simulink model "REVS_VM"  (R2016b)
settings: Solver=ode3  StartTime=REVS.sim_start_time_secs  StopTime=Inf  FixedStep=REVS.sim_step_time_secs  MaxStep=REVS.sim_step_time_secs  EnableMultiTasking=on
StopFcn:
  | postproc_datalog;
  | postproc_audit;
  | postproc_result;
model workspace (MATLAB code in the model file):
  other statements: REVS_setup_variants
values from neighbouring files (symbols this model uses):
  accessory = class_accessory_data    [class_test_data.m]
  battery = class_battery_data    [class_accessory_data.m]    (also in class_REVS_electric.m = class_REVS_battery)
  brake = struct(	'max_torque_Nm',[], 						'proportion_norm',1.0, 						'inertia_kgm2',0.0)    [class_REVS_drive_axle.m]
  engine = class_engine_data    [class_test_data.m]
  final_drive = struct(	'gear_ratio',[], 								'efficiency_norm',[], 								'inertia_kgm2',[] )    [class_REVS_drive_axle.m]
  gear = class_REVS_gearbox    [class_REVS_AT_transmission.m]
  tire = struct(	'radius_m',[], 						'rolling_resistance_coefficient',0, 						'vehicle_weight_norm',1.0,  						'wheel_slip_torque_Nm',[],  						'inertia_kgm2',0.0)    [class_REVS_drive_axle.m]
  torque_converter = class_REVS_torque_converter    [class_REVS_AT_transmission.m]
  transmission = class_transmission_data    [class_test_data.m]
  vehicle = class_vehicle_data    [class_test_data.m]
undefined symbols (not defined in the file or in its folder): alternator, ambient, controls, convert, DelayTimeSecs, drive_cycle, driver, electric, gear_strategy, InitialCondition, InitialValue, LoadSource, LookupStructure, MultiplyPosInputs, Normalize, NumPhases, REVS, SpeedSource, starter, tableshift, UpperSaturationLimit, Value, VerboseLevel, VerboseSignal
libraries: simulink x153
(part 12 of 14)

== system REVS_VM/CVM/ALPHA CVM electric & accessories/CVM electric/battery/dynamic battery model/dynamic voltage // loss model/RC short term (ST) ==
  bus_in : Inport
  Add2 : Sum  Inputs=+-
  Bus Selector : BusSelector  OutputSignals=pack_curr_A
  Cp short term : Subsystem
  Integrator : Integrator
  Product4 : Product  Inputs=*/
  Product5 : Product  Inputs=*/
  Rp short term : Subsystem
  to datalog with base name : Subsystem
  to datalog with base name1 : Subsystem
  to datalog with base name2 : Subsystem
  RC_ST_V : Outport
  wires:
  Rp short term/1(Rp_ST_Ohm) -> to datalog with base name1/1(Var), Product5/2
  Bus Selector/1 -> Add2/1  "<pack_curr_A>"
  Integrator/1 -> RC_ST_V/1, to datalog with base name/1(Var), Product5/1
  Product4/1 -> Integrator/1
  Product5/1 -> Add2/2  "I ST"
  Add2/1 -> Product4/1
  Cp short term/1(Cp_ST_Farad) -> to datalog with base name2/1(Var), Product4/2
  bus_in/1 -> Cp short term/1(bus_in), Bus Selector/1, Rp short term/1(bus_in)

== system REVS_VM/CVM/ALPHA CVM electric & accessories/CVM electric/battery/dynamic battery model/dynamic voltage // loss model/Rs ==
  bus_in : Inport
  Bus Selector1 : BusSelector  OutputSignals=pack_curr_A
  Product1 : Product
  Rs charge : Subsystem
  Rs discharge : Subsystem
  Switch : Switch  Criteria=u2 > Threshold
  to datalog with base name : Subsystem
  to datalog with base name1 : Subsystem
  Rs_V : Outport
  Rs_dis_Ohm : Outport  Port=2
  Rs_chg_Ohm : Outport  Port=3
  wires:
  Product1/1 -> Rs_V/1, to datalog with base name/1(Var)
  Switch/1 -> Product1/2, to datalog with base name1/1(Var)
  Rs discharge/1(out) -> Switch/1, Rs_dis_Ohm/1
  Rs charge/1(out) -> Rs_chg_Ohm/1, Switch/3
  Bus Selector1/1 -> Product1/1, Switch/2  "<pack_curr_A>"
  bus_in/1 -> Rs discharge/1(bus), Rs charge/1(bus), Bus Selector1/1

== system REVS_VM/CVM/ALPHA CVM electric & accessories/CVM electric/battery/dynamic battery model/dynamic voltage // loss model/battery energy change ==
  Var : Inport
  Compare To Constant : simulink/Logic and Bit Operations/Compare To Constant  relop=>=  const=1  OutDataTypeStr=boolean
  Constant : Constant  Value=VerboseSignal
  Subsystem : Subsystem
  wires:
  Constant/1 -> Compare To Constant/1
  Compare To Constant/1 -> Subsystem/Enable
  Var/1 -> Subsystem/1(In1)

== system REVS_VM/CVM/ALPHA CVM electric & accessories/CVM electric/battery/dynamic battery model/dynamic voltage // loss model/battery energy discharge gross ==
  Var : Inport
  Compare To Constant : simulink/Logic and Bit Operations/Compare To Constant  relop=>=  const=1  OutDataTypeStr=boolean
  Constant : Constant  Value=VerboseSignal
  Subsystem : Subsystem
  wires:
  Constant/1 -> Compare To Constant/1
  Compare To Constant/1 -> Subsystem/Enable
  Var/1 -> Subsystem/1(In1)

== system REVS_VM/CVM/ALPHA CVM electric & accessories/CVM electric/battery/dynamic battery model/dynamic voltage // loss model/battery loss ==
  Var : Inport
  Compare To Constant : simulink/Logic and Bit Operations/Compare To Constant  relop=>=  const=1  OutDataTypeStr=boolean
  Constant : Constant  Value=VerboseSignal
  Subsystem : Subsystem
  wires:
  Constant/1 -> Compare To Constant/1
  Compare To Constant/1 -> Subsystem/Enable
  Var/1 -> Subsystem/1(In1)

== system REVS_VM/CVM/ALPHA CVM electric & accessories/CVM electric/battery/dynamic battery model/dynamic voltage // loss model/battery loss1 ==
  Var : Inport
  Compare To Constant : simulink/Logic and Bit Operations/Compare To Constant  relop=>=  const=1  OutDataTypeStr=boolean
  Constant : Constant  Value=VerboseSignal
  Subsystem : Subsystem
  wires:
  Constant/1 -> Compare To Constant/1
  Compare To Constant/1 -> Subsystem/Enable
  Var/1 -> Subsystem/1(In1)

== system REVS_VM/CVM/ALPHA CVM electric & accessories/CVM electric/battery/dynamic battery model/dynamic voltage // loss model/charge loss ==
  charge_eff_norm : Inport
  pack_curr_A : Inport  Port=2
  OCV_V : Inport  Port=3
  Compare To Zero : simulink/Logic and Bit Operations/Compare To Zero  relop=<=  OutDataTypeStr=uint8
  Constant2 : Constant
  Data Type Conversion : DataTypeConversion  OutDataTypeStr=double
  Gain1 : Gain  Gain=-1
  Product7 : Product  Inputs=4  OutDataTypeStr=double
  Sum : Sum  Inputs=|+-
  chg_loss_pwr_W : Outport
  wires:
  Gain1/1 -> Product7/3
  pack_curr_A/1 -> Gain1/1, Compare To Zero/1
  OCV_V/1 -> Product7/4
  charge_eff_norm/1 -> Sum/2
  Data Type Conversion/1 -> Product7/2
  Constant2/1 -> Sum/1
  Compare To Zero/1 -> Data Type Conversion/1
  Sum/1 -> Product7/1
  Product7/1 -> chg_loss_pwr_W/1

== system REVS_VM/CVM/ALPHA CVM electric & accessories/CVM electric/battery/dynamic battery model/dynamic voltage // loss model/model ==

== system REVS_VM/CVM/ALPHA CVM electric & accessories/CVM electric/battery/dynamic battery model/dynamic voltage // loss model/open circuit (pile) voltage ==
  bus_in : Inport
  Add : Sum
  Bus Selector : BusSelector  OutputSignals=pack_curr_A
  Gain : Gain  Gain=0.5
  OCV charge dynamic : Subsystem
  OCV discharge dynamic : Subsystem
  Switch : Switch  Criteria=u2 ~= 0
  Switch1 : Switch
  to datalog with base name : Subsystem
  use average : Constant  Value=battery.use_average_open_circuit_Volts
  OCV_V : Outport
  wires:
  Switch/1 -> OCV_V/1, to datalog with base name/1(Var)
  OCV discharge dynamic/1(out) -> Add/1, Switch1/1
  OCV charge dynamic/1(out) -> Add/2, Switch1/3
  Switch1/1 -> Switch/3
  use average/1 -> Switch/2
  bus_in/1 -> OCV discharge dynamic/1(bus), OCV charge dynamic/1(bus), Bus Selector/1
  Add/1 -> Gain/1
  Gain/1 -> Switch/1
  Bus Selector/1 -> Switch1/2  "<pack_curr_A>"

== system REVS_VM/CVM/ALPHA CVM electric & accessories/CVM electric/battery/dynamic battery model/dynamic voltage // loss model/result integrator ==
  in : Inport
  Data Type Conversion : DataTypeConversion  OutDataTypeStr=double
  Integrator1 : Integrator  UpperSaturationLimit=Inf  LowerSaturationLimit=0  ZeroCross=off
  Integrator2 : Integrator  UpperSaturationLimit=Inf  LowerSaturationLimit=0  ZeroCross=off
  Phase To Workspace : ToWorkspace  VariableName=result__phase_battery_delta_kJ  SampleTime=-1
  Product1 : Product  Multiplication=Matrix(*)
  Reshape : Reshape
  Total To Workspace : ToWorkspace  VariableName=result__total_battery_delta_kJ  SampleTime=-1
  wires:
  Reshape/1 -> Integrator1/1, Product1/1
  Data Type Conversion/1 -> Reshape/1
  Integrator2/1 -> Phase To Workspace/1
  [REVS_phase_flag] -> Product1/2
  Product1/1 -> Integrator2/1
  Integrator1/1 -> Total To Workspace/1
  in/1 -> Data Type Conversion/1

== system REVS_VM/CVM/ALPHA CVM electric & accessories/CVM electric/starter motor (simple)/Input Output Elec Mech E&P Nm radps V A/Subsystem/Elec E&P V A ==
  volts_V : Inport
  curr_A : Inport  Port=2
  Compare To Constant : simulink/Logic and Bit Operations/Compare To Constant  relop=>=  const=1  OutDataTypeStr=boolean
  Constant : Constant  Value=VerboseSignal
  Subsystem : Subsystem
  pos_kJ : Outport
  neg_kJ : Outport  Port=2
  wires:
  volts_V/1 -> Subsystem/1(volts_V)
  curr_A/1 -> Subsystem/2(curr_A)
  Subsystem/1(pos_kJ) -> pos_kJ/1
  Subsystem/2(neg_kJ) -> neg_kJ/1
  Compare To Constant/1 -> Subsystem/Enable
  Constant/1 -> Compare To Constant/1

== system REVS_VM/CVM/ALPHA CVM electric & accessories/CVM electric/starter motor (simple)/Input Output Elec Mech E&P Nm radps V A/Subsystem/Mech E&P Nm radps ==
  " trq_Nm" : Inport
  spd_radps : Inport  Port=2
  iner_kgm2 : Inport  Port=3
  Compare To Constant : simulink/Logic and Bit Operations/Compare To Constant  relop=>=  const=1  OutDataTypeStr=boolean
  Constant : Constant  Value=VerboseSignal
  Subsystem : Subsystem
  pos_kJ : Outport
  neg_kJ : Outport  Port=2
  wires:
  " trq_Nm"/1 -> Subsystem/1(" trq_Nm")
  spd_radps/1 -> Subsystem/2(spd_radps)
  iner_kgm2/1 -> Subsystem/3(iner_kgm2)
  Compare To Constant/1 -> Subsystem/Enable
  Subsystem/1(pos_kJ) -> pos_kJ/1
  Subsystem/2(neg_kJ) -> neg_kJ/1
  Constant/1 -> Compare To Constant/1

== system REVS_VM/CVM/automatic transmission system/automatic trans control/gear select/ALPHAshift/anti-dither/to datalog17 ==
  Var : Inport
  Constant : Constant  Value=VerboseSignal
  Constant1 : Constant  Value=VerboseLevel
  Relational Operator : RelationalOperator  OutDataTypeStr=boolean  ZeroCross=off
  Subsystem : Subsystem
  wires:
  Constant1/1 -> Relational Operator/2
  Constant/1 -> Relational Operator/1
  Relational Operator/1 -> Subsystem/Enable
  Var/1 -> Subsystem/1(In1)

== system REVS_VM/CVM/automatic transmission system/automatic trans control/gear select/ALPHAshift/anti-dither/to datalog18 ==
  Var : Inport
  Constant : Constant  Value=VerboseSignal
  Constant1 : Constant  Value=VerboseLevel
  Relational Operator : RelationalOperator  OutDataTypeStr=boolean  ZeroCross=off
  Subsystem : Subsystem
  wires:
  Constant1/1 -> Relational Operator/2
  Constant/1 -> Relational Operator/1
  Relational Operator/1 -> Subsystem/Enable
  Var/1 -> Subsystem/1(In1)

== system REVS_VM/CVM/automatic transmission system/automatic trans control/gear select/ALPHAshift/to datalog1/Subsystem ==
  In1 : Inport
  Enable : EnablePort
  To Workspace : ToWorkspace  VariableName=datalog__ALPHAshift__desired_gear_num  SampleTime=-1
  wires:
  In1/1 -> To Workspace/1

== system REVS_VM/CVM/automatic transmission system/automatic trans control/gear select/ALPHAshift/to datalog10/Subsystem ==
  In1 : Inport
  Enable : EnablePort
  To Workspace : ToWorkspace  VariableName=datalog__ALPHAshift__kickdown_timer  SampleTime=-1
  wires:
  In1/1 -> To Workspace/1

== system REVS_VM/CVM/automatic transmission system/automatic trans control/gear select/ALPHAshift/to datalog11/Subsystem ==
  In1 : Inport
  Enable : EnablePort
  To Workspace : ToWorkspace  VariableName=datalog__ALPHAshift__kickdown_ratio  SampleTime=-1
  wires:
  In1/1 -> To Workspace/1

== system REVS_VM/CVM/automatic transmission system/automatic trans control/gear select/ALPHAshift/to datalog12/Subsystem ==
  In1 : Inport
  Enable : EnablePort
  To Workspace : ToWorkspace  VariableName=datalog__ALPHAshift__shift_delay_timer  SampleTime=-1
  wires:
  In1/1 -> To Workspace/1

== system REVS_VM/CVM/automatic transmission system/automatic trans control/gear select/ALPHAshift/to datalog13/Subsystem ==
  In1 : Inport
  Enable : EnablePort
  To Workspace : ToWorkspace  VariableName=datalog__ALPHAshift__in_gear_timer  SampleTime=-1
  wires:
  In1/1 -> To Workspace/1

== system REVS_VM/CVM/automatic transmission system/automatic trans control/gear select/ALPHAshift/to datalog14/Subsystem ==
  In1 : Inport
  Enable : EnablePort
  To Workspace : ToWorkspace  VariableName=datalog__ALPHAshift__gear_avail_torque_Nm  SampleTime=-1
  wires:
  In1/1 -> To Workspace/1

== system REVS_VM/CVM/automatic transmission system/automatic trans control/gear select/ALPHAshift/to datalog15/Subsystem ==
  In1 : Inport
  Enable : EnablePort
  To Workspace : ToWorkspace  VariableName=datalog__ALPHAshift__gear_speed_radps  SampleTime=-1
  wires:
  In1/1 -> To Workspace/1

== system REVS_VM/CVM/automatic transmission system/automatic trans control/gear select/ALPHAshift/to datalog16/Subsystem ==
  In1 : Inport
  Enable : EnablePort
  To Workspace : ToWorkspace  VariableName=datalog__ALPHAshift__gear_torque_Nm  SampleTime=-1
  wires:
  In1/1 -> To Workspace/1

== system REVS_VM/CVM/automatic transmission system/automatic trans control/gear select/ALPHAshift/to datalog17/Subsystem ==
  In1 : Inport
  Enable : EnablePort
  To Workspace : ToWorkspace  VariableName=datalog__ALPHAshift__gear_cost  SampleTime=-1
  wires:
  In1/1 -> To Workspace/1

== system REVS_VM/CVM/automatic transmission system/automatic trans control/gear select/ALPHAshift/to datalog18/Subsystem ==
  In1 : Inport
  Enable : EnablePort
  To Workspace : ToWorkspace  VariableName=datalog__ALPHAshift__kickdown_disability_code  SampleTime=-1
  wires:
  In1/1 -> To Workspace/1

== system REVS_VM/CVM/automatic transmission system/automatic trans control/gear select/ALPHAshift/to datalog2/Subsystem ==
  In1 : Inport
  Enable : EnablePort
  To Workspace : ToWorkspace  VariableName=datalog__ALPHAshift__shift_reason  SampleTime=-1
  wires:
  In1/1 -> To Workspace/1

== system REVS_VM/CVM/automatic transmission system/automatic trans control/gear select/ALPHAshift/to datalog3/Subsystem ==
  In1 : Inport
  Enable : EnablePort
  To Workspace : ToWorkspace  VariableName=datalog__ALPHAshift__disability_code  SampleTime=-1
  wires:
  In1/1 -> To Workspace/1

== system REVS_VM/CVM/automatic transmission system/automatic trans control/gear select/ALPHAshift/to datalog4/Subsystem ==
  In1 : Inport
  Enable : EnablePort
  To Workspace : ToWorkspace  VariableName=datalog__ALPHAshift__current_gear_num  SampleTime=-1
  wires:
  In1/1 -> To Workspace/1

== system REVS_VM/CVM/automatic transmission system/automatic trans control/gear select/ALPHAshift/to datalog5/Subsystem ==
  In1 : Inport
  Enable : EnablePort
  To Workspace : ToWorkspace  VariableName=datalog__ALPHAshift__gear_available  SampleTime=-1
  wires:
  In1/1 -> To Workspace/1

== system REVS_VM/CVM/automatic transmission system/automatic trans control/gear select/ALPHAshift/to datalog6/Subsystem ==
  In1 : Inport
  Enable : EnablePort
  To Workspace : ToWorkspace  VariableName=datalog__ALPHAshift__shift_type  SampleTime=-1
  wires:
  In1/1 -> To Workspace/1

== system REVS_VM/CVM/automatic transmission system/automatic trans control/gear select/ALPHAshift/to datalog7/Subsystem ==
  In1 : Inport
  Enable : EnablePort
  To Workspace : ToWorkspace  VariableName=datalog__ALPHAshift__better_fuel_gear  SampleTime=-1
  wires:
  In1/1 -> To Workspace/1

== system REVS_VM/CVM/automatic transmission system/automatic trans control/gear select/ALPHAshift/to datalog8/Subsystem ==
  In1 : Inport
  Enable : EnablePort
  To Workspace : ToWorkspace  VariableName=datalog__ALPHAshift__min_fuel_gear  SampleTime=-1
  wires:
  In1/1 -> To Workspace/1

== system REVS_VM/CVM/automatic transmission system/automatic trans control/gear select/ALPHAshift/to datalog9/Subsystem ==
  In1 : Inport
  Enable : EnablePort
  To Workspace : ToWorkspace  VariableName=datalog__ALPHAshift__desired_shift_reason  SampleTime=-1
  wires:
  In1/1 -> To Workspace/1

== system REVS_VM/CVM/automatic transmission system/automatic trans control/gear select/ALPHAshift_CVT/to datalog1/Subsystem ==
  In1 : Inport
  Enable : EnablePort
  To Workspace : ToWorkspace  VariableName=datalog__cvtshift__target_ratio  SampleTime=-1
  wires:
  In1/1 -> To Workspace/1

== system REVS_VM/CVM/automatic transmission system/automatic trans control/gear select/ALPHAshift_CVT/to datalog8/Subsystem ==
  In1 : Inport
  Enable : EnablePort
  To Workspace : ToWorkspace  VariableName=datalog__cvtshift__target_speed_radps  SampleTime=-1
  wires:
  In1/1 -> To Workspace/1

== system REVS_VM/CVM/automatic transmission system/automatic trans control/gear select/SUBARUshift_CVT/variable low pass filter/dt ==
  Clock : Clock
  Memory1 : Memory
  Sum : Sum  Inputs=|-+
  dt : Outport
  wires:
  Clock/1 -> Sum/2, Memory1/1
  Memory1/1 -> Sum/1
  Sum/1 -> dt/1

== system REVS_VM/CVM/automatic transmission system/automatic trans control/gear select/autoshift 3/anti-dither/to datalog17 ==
  Var : Inport
  Constant : Constant  Value=VerboseSignal
  Constant1 : Constant  Value=VerboseLevel
  Relational Operator : RelationalOperator  OutDataTypeStr=boolean  ZeroCross=off
  Subsystem : Subsystem
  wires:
  Constant1/1 -> Relational Operator/2
  Constant/1 -> Relational Operator/1
  Relational Operator/1 -> Subsystem/Enable
  Var/1 -> Subsystem/1(In1)

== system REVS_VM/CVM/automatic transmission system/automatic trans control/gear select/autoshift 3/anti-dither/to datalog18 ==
  Var : Inport
  Constant : Constant  Value=VerboseSignal
  Constant1 : Constant  Value=VerboseLevel
  Relational Operator : RelationalOperator  OutDataTypeStr=boolean  ZeroCross=off
  Subsystem : Subsystem
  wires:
  Constant1/1 -> Relational Operator/2
  Constant/1 -> Relational Operator/1
  Relational Operator/1 -> Subsystem/Enable
  Var/1 -> Subsystem/1(In1)

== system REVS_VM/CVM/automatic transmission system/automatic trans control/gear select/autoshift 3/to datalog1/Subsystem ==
  In1 : Inport
  Enable : EnablePort
  To Workspace : ToWorkspace  VariableName=datalog__autoshift3__desired_gear_num  SampleTime=-1
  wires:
  In1/1 -> To Workspace/1

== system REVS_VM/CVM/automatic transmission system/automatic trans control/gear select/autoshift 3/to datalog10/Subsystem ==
  In1 : Inport
  Enable : EnablePort
  To Workspace : ToWorkspace  VariableName=datalog__autoshift3__kickdown_timer  SampleTime=-1
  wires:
  In1/1 -> To Workspace/1

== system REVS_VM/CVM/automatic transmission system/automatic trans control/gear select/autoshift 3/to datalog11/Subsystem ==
  In1 : Inport
  Enable : EnablePort
  To Workspace : ToWorkspace  VariableName=datalog__autoshift3__kickdown_ratio  SampleTime=-1
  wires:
  In1/1 -> To Workspace/1

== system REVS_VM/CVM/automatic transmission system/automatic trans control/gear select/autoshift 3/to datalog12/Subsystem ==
  In1 : Inport
  Enable : EnablePort
  To Workspace : ToWorkspace  VariableName=datalog__autoshift3__shift_delay_timer  SampleTime=-1
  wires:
  In1/1 -> To Workspace/1

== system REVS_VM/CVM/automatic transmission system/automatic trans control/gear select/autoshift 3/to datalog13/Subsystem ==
  In1 : Inport
  Enable : EnablePort
  To Workspace : ToWorkspace  VariableName=datalog__autoshift3__in_gear_timer  SampleTime=-1
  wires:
  In1/1 -> To Workspace/1

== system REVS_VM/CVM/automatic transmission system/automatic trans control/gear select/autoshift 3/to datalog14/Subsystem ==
  In1 : Inport
  Enable : EnablePort
  To Workspace : ToWorkspace  VariableName=datalog__autoshift3__gear_avail_torque_Nm  SampleTime=-1
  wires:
  In1/1 -> To Workspace/1

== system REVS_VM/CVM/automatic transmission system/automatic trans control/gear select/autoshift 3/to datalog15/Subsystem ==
  In1 : Inport
  Enable : EnablePort
  To Workspace : ToWorkspace  VariableName=datalog__autoshift3__gear_speed_radps  SampleTime=-1
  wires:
  In1/1 -> To Workspace/1

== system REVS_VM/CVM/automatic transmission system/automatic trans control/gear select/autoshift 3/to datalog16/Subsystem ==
  In1 : Inport
  Enable : EnablePort
  To Workspace : ToWorkspace  VariableName=datalog__autoshift3__gear_torque_Nm  SampleTime=-1
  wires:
  In1/1 -> To Workspace/1

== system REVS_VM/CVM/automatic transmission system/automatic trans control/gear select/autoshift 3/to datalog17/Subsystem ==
  In1 : Inport
  Enable : EnablePort
  To Workspace : ToWorkspace  VariableName=datalog__autoshift3__gear_cost  SampleTime=-1
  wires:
  In1/1 -> To Workspace/1

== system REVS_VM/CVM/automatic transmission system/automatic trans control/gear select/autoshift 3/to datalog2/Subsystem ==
  In1 : Inport
  Enable : EnablePort
  To Workspace : ToWorkspace  VariableName=datalog__autoshift3__shift_reason  SampleTime=-1
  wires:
  In1/1 -> To Workspace/1

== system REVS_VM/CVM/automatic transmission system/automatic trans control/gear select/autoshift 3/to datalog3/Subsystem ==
  In1 : Inport
  Enable : EnablePort
  To Workspace : ToWorkspace  VariableName=datalog__autoshift3__disability_code  SampleTime=-1
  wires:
  In1/1 -> To Workspace/1

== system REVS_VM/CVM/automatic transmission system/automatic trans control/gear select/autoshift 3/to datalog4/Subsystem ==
  In1 : Inport
  Enable : EnablePort
  To Workspace : ToWorkspace  VariableName=datalog__autoshift3__current_gear_num  SampleTime=-1
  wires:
  In1/1 -> To Workspace/1

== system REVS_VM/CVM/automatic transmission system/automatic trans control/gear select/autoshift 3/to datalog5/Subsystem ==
  In1 : Inport
  Enable : EnablePort
  To Workspace : ToWorkspace  VariableName=datalog__autoshift3__gear_available  SampleTime=-1
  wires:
  In1/1 -> To Workspace/1

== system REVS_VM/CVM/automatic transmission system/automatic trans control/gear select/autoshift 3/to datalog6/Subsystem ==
  In1 : Inport
  Enable : EnablePort
  To Workspace : ToWorkspace  VariableName=datalog__autoshift3__shift_type  SampleTime=-1
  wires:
  In1/1 -> To Workspace/1

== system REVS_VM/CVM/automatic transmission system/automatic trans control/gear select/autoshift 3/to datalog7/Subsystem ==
  In1 : Inport
  Enable : EnablePort
  To Workspace : ToWorkspace  VariableName=datalog__autoshift3__better_fuel_gear  SampleTime=-1
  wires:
  In1/1 -> To Workspace/1

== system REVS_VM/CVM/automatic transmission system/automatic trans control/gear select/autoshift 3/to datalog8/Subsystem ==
  In1 : Inport
  Enable : EnablePort
  To Workspace : ToWorkspace  VariableName=datalog__autoshift3__min_fuel_gear  SampleTime=-1
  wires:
  In1/1 -> To Workspace/1

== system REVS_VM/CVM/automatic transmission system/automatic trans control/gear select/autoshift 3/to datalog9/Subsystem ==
  In1 : Inport
  Enable : EnablePort
  To Workspace : ToWorkspace  VariableName=datalog__autoshift3__desired_shift_reason  SampleTime=-1
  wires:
  In1/1 -> To Workspace/1

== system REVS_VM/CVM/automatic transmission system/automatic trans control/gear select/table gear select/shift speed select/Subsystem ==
  veh_spd_mps : Inport
  Axle Speed (rad/sec) : Product  Inputs=/*
  Non Zero : Saturate  UpperLimit=Inf  LowerLimit=eps  ZeroCross=off
  Tire Radius (m) : Constant  Value=vehicle.drive_axle1.tire.radius_m
  wheel_spd_radps : Outport
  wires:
  veh_spd_mps/1 -> Axle Speed (rad/sec)/2
  Non Zero/1 -> Axle Speed (rad/sec)/1
  Axle Speed (rad/sec)/1 -> wheel_spd_radps/1
  Tire Radius (m)/1 -> Non Zero/1

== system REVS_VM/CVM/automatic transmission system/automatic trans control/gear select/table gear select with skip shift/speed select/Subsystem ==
  veh_spd_mps : Inport
  Axle Speed (rad/sec) : Product  Inputs=/*
  Non Zero : Saturate  UpperLimit=Inf  LowerLimit=eps  ZeroCross=off
  Tire Radius (m) : Constant  Value=vehicle.drive_axle1.tire.radius_m
  wheel_spd_radps : Outport
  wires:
  veh_spd_mps/1 -> Axle Speed (rad/sec)/2
  Non Zero/1 -> Axle Speed (rad/sec)/1
  Axle Speed (rad/sec)/1 -> wheel_spd_radps/1
  Tire Radius (m)/1 -> Non Zero/1

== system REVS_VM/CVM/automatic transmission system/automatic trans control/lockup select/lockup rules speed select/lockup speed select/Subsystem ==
  veh_spd_mps : Inport
  Axle Speed (rad/sec) : Product  Inputs=/*
  Non Zero : Saturate  UpperLimit=Inf  LowerLimit=eps  ZeroCross=off
  Tire Radius (m) : Constant  Value=vehicle.drive_axle1.tire.radius_m
  wheel_spd_radps : Outport
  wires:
  veh_spd_mps/1 -> Axle Speed (rad/sec)/2
  Non Zero/1 -> Axle Speed (rad/sec)/1
  Axle Speed (rad/sec)/1 -> wheel_spd_radps/1
  Tire Radius (m)/1 -> Non Zero/1

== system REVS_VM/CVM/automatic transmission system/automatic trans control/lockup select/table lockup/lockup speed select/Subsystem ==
  veh_spd_mps : Inport
  Axle Speed (rad/sec) : Product  Inputs=/*
  Non Zero : Saturate  UpperLimit=Inf  LowerLimit=eps  ZeroCross=off
  Tire Radius (m) : Constant  Value=vehicle.drive_axle1.tire.radius_m
  wheel_spd_radps : Outport
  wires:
  veh_spd_mps/1 -> Axle Speed (rad/sec)/2
  Non Zero/1 -> Axle Speed (rad/sec)/1
  Axle Speed (rad/sec)/1 -> wheel_spd_radps/1
  Tire Radius (m)/1 -> Non Zero/1

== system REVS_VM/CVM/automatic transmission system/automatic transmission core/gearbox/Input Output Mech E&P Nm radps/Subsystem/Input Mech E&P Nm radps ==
  " trq_Nm" : Inport
  spd_radps : Inport  Port=2
  iner_kgm2 : Inport  Port=3
  Compare To Constant : simulink/Logic and Bit Operations/Compare To Constant  relop=>=  const=1  OutDataTypeStr=boolean
  Constant : Constant  Value=VerboseSignal
  Subsystem : Subsystem
  pos_kJ : Outport
  neg_kJ : Outport  Port=2
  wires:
  " trq_Nm"/1 -> Subsystem/1(" trq_Nm")
  spd_radps/1 -> Subsystem/2(spd_radps)
  iner_kgm2/1 -> Subsystem/3(iner_kgm2)
  Compare To Constant/1 -> Subsystem/Enable
  Subsystem/1(pos_kJ) -> pos_kJ/1
  Subsystem/2(neg_kJ) -> neg_kJ/1
  Constant/1 -> Compare To Constant/1

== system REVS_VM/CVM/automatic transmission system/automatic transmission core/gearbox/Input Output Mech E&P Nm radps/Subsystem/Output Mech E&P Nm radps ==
  " trq_Nm" : Inport
  spd_radps : Inport  Port=2
  iner_kgm2 : Inport  Port=3
  Compare To Constant : simulink/Logic and Bit Operations/Compare To Constant  relop=>=  const=1  OutDataTypeStr=boolean
  Constant : Constant  Value=VerboseSignal
  Subsystem : Subsystem
  pos_kJ : Outport
  neg_kJ : Outport  Port=2
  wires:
  " trq_Nm"/1 -> Subsystem/1(" trq_Nm")
  spd_radps/1 -> Subsystem/2(spd_radps)
  iner_kgm2/1 -> Subsystem/3(iner_kgm2)
  Compare To Constant/1 -> Subsystem/Enable
  Subsystem/1(pos_kJ) -> pos_kJ/1
  Subsystem/2(neg_kJ) -> neg_kJ/1
  Constant/1 -> Compare To Constant/1

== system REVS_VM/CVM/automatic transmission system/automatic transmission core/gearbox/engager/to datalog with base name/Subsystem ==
  Var : Inport
  Enable : EnablePort
  To Workspace : ToWorkspace  VariableName=datalog__gearbox__current_gear  SampleTime=-1
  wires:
  Var/1 -> To Workspace/1

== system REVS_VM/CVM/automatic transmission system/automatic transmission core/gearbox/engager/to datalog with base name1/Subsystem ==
  Var : Inport
  Enable : EnablePort
  To Workspace : ToWorkspace  VariableName=datalog__gearbox__gearbox__engage_norm  SampleTime=-1
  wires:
  Var/1 -> To Workspace/1

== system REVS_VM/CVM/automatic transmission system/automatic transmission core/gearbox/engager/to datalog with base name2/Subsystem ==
  Var : Inport
  Enable : EnablePort
  To Workspace : ToWorkspace  VariableName=datalog__gearbox__command_gear  SampleTime=-1
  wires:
  Var/1 -> To Workspace/1

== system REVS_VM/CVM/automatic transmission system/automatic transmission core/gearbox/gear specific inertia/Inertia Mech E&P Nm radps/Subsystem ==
  trq_Nm : Inport
  spd_radps : Inport  Port=2
  Enable : EnablePort  ZeroCross=off
  Mech Energy Nm radps : Subsystem  TreatAsAtomicUnit=on
  energy_to_workspace : ToWorkspace  VariableName=audit__mech__gearbox__inertia_spinup_loss_kJ  SampleTime=-1
  neg_energy_to_workspace : ToWorkspace  VariableName=audit__mech__gearbox__inertia_spinup_loss_neg_kJ  SampleTime=-1
  pos_energy_to_workspace : ToWorkspace  VariableName=audit__mech__gearbox__inertia_spinup_loss_pos_kJ  SampleTime=-1
  power_to_workspace : ToWorkspace  VariableName=audit__mech__gearbox__inertia_spinup_loss_kW  SampleTime=-1
  speed_to_workspace : ToWorkspace  VariableName=audit__mech__gearbox__inertia_spinup_loss_radps  SampleTime=-1
  torque_to_workspace : ToWorkspace  VariableName=audit__mech__gearbox__inertia_spinup_loss_Nm  SampleTime=-1
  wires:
  Mech Energy Nm radps/1("total_kJ ") -> energy_to_workspace/1
  Mech Energy Nm radps/4(pwr_kW) -> power_to_workspace/1
  Mech Energy Nm radps/2("pos_kJ ") -> pos_energy_to_workspace/1
  Mech Energy Nm radps/3(neg_kJ) -> neg_energy_to_workspace/1
  trq_Nm/1 -> torque_to_workspace/1, Mech Energy Nm radps/1(trq_Nm)
  spd_radps/1 -> speed_to_workspace/1, Mech Energy Nm radps/2(spd_radps)

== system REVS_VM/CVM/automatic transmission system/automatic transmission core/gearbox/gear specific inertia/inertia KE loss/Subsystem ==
  In1 : Inport
  Enable : EnablePort
  To Workspace : ToWorkspace  VariableName=audit__mech__gearbox__inertia_KE_loss_kJ  SampleTime=-1
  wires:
  In1/1 -> To Workspace/1

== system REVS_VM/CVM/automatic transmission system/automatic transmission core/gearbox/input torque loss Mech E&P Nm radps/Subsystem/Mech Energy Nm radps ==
  trq_Nm : Inport
  spd_radps : Inport  Port=2
  Gain : Gain  Gain=-1
  Integrator : Integrator  ZeroCross=off
  Integrator1 : Integrator  ZeroCross=off
  Integrator2 : Integrator  ZeroCross=off
  Mux : Mux  Inputs=2
  Neg : Fcn  Expr=u(1)*(u(1) <= 0)
  Pos : Fcn  Expr=u(1)*(u(1) >= 0)
  calc_Power_kW : Fcn  Expr=u(1)*u(2)/1000
  "total_kJ " : Outport
  "pos_kJ " : Outport  Port=2
  neg_kJ : Outport  Port=3
  pwr_kW : Outport  Port=4
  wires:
  calc_Power_kW/1 -> Pos/1, Neg/1, pwr_kW/1, Integrator/1
  Gain/1 -> neg_kJ/1
  Integrator1/1 -> "pos_kJ "/1
  Integrator2/1 -> Gain/1
  Neg/1 -> Integrator2/1
  Pos/1 -> Integrator1/1
  spd_radps/1 -> Mux/2
  trq_Nm/1 -> Mux/1
  Mux/1 -> calc_Power_kW/1
  Integrator/1 -> "total_kJ "/1

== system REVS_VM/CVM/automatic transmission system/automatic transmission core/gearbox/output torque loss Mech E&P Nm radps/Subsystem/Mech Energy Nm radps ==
  trq_Nm : Inport
  spd_radps : Inport  Port=2
  Gain : Gain  Gain=-1
  Integrator : Integrator  ZeroCross=off
  Integrator1 : Integrator  ZeroCross=off
  Integrator2 : Integrator  ZeroCross=off
  Mux : Mux  Inputs=2
  Neg : Fcn  Expr=u(1)*(u(1) <= 0)
  Pos : Fcn  Expr=u(1)*(u(1) >= 0)
  calc_Power_kW : Fcn  Expr=u(1)*u(2)/1000
  "total_kJ " : Outport
  "pos_kJ " : Outport  Port=2
  neg_kJ : Outport  Port=3
  pwr_kW : Outport  Port=4
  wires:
  calc_Power_kW/1 -> Pos/1, Neg/1, pwr_kW/1, Integrator/1
  Gain/1 -> neg_kJ/1
  Integrator1/1 -> "pos_kJ "/1
  Integrator2/1 -> Gain/1
  Neg/1 -> Integrator2/1
  Pos/1 -> Integrator1/1
  spd_radps/1 -> Mux/2
  trq_Nm/1 -> Mux/1
  Mux/1 -> calc_Power_kW/1
  Integrator/1 -> "total_kJ "/1

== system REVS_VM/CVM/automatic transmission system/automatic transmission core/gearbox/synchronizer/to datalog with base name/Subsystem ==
  Var : Inport
  Enable : EnablePort
  To Workspace : ToWorkspace  VariableName=datalog__gearbox__gear_synchronizer_lockup  SampleTime=-1
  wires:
  Var/1 -> To Workspace/1

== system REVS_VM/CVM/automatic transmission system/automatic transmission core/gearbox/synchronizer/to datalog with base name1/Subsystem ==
  Var : Inport
  Enable : EnablePort
  To Workspace : ToWorkspace  VariableName=datalog__gearbox__synchronizer_transmit_torque_Nm  SampleTime=-1
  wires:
  Var/1 -> To Workspace/1

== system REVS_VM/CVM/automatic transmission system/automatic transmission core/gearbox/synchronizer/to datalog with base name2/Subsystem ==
  Var : Inport
  Enable : EnablePort
  To Workspace : ToWorkspace  VariableName=datalog__gearbox__synchronizer_engage_torque_Nm  SampleTime=-1
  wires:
  Var/1 -> To Workspace/1

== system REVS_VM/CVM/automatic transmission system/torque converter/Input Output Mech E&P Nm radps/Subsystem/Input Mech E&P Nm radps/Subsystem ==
  " trq_Nm" : Inport
  spd_radps : Inport  Port=2
  iner_kgm2 : Inport  Port=3
  Enable : EnablePort  ZeroCross=off
  KE_to_workspace : ToWorkspace  VariableName=audit__mech__torque_converter__input_KE_kJ  SampleTime=-1
  Mech Energy Nm radps : Subsystem  TreatAsAtomicUnit=on
  Mult : Product  Inputs=**
  Square : Math  Operator=square
  energy_to_workspace : ToWorkspace  VariableName=audit__mech__torque_converter__input_kJ  SampleTime=-1
  inertia_to_workspace : ToWorkspace  VariableName=audit__mech__torque_converter__input_kgm2  SampleTime=-1
  neg_energy_to_workspace : ToWorkspace  VariableName=audit__mech__torque_converter__input_neg_kJ  SampleTime=-1
  one half : Gain  Gain=0.5/1000
  pos_energy_to_workspace : ToWorkspace  VariableName=audit__mech__torque_converter__input_pos_kJ  SampleTime=-1
  power_to_workspace : ToWorkspace  VariableName=audit__mech__torque_converter__input_kW  SampleTime=-1
  speed_to_workspace : ToWorkspace  VariableName=audit__mech__torque_converter__input_radps  SampleTime=-1
  torque_to_workspace : ToWorkspace  VariableName=audit__mech__torque_converter__input_Nm  SampleTime=-1
  pos_kJ : Outport  InitialOutput=0
  neg_kJ : Outport  Port=2  InitialOutput=0
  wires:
  Mult/1 -> one half/1
  Square/1 -> Mult/1
  one half/1 -> KE_to_workspace/1
  Mech Energy Nm radps/4(pwr_kW) -> power_to_workspace/1
  Mech Energy Nm radps/1("total_kJ ") -> energy_to_workspace/1
  iner_kgm2/1 -> inertia_to_workspace/1, Mult/2
  spd_radps/1 -> Mech Energy Nm radps/2(spd_radps), speed_to_workspace/1, Square/1
  " trq_Nm"/1 -> Mech Energy Nm radps/1(trq_Nm), torque_to_workspace/1
  Mech Energy Nm radps/2("pos_kJ ") -> pos_kJ/1, pos_energy_to_workspace/1
  Mech Energy Nm radps/3(neg_kJ) -> neg_energy_to_workspace/1, neg_kJ/1

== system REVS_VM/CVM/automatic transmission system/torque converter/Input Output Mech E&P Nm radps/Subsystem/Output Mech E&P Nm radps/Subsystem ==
  " trq_Nm" : Inport
  spd_radps : Inport  Port=2
  iner_kgm2 : Inport  Port=3
  Enable : EnablePort  ZeroCross=off
  KE_to_workspace : ToWorkspace  VariableName=audit__mech__torque_converter__output_KE_kJ  SampleTime=-1
  Mech Energy Nm radps : Subsystem  TreatAsAtomicUnit=on
  Mult : Product  Inputs=**
  Square : Math  Operator=square
  energy_to_workspace : ToWorkspace  VariableName=audit__mech__torque_converter__output_kJ  SampleTime=-1
  inertia_to_workspace : ToWorkspace  VariableName=audit__mech__torque_converter__output_kgm2  SampleTime=-1
  neg_energy_to_workspace : ToWorkspace  VariableName=audit__mech__torque_converter__output_neg_kJ  SampleTime=-1
  one half : Gain  Gain=0.5/1000
  pos_energy_to_workspace : ToWorkspace  VariableName=audit__mech__torque_converter__output_pos_kJ  SampleTime=-1
  power_to_workspace : ToWorkspace  VariableName=audit__mech__torque_converter__output_kW  SampleTime=-1
  speed_to_workspace : ToWorkspace  VariableName=audit__mech__torque_converter__output_radps  SampleTime=-1
  torque_to_workspace : ToWorkspace  VariableName=audit__mech__torque_converter__output_Nm  SampleTime=-1
  pos_kJ : Outport  InitialOutput=0
  neg_kJ : Outport  Port=2  InitialOutput=0
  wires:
  Mult/1 -> one half/1
  Square/1 -> Mult/1
  one half/1 -> KE_to_workspace/1
  Mech Energy Nm radps/4(pwr_kW) -> power_to_workspace/1
  Mech Energy Nm radps/1("total_kJ ") -> energy_to_workspace/1
  iner_kgm2/1 -> inertia_to_workspace/1, Mult/2
  spd_radps/1 -> Mech Energy Nm radps/2(spd_radps), speed_to_workspace/1, Square/1
  " trq_Nm"/1 -> Mech Energy Nm radps/1(trq_Nm), torque_to_workspace/1
  Mech Energy Nm radps/2("pos_kJ ") -> pos_kJ/1, pos_energy_to_workspace/1
  Mech Energy Nm radps/3(neg_kJ) -> neg_energy_to_workspace/1, neg_kJ/1

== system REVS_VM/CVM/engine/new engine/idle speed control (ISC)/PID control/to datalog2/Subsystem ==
  In1 : Inport
  Enable : EnablePort
  To Workspace : ToWorkspace  VariableName=datalog__engine__ISC_Ki_torque_Nm  SampleTime=-1
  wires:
  In1/1 -> To Workspace/1

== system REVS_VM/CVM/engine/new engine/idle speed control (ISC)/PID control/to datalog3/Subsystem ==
  In1 : Inport
  Enable : EnablePort
  To Workspace : ToWorkspace  VariableName=datalog__engine__ISC_Kp_torque_Nm  SampleTime=-1
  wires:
  In1/1 -> To Workspace/1

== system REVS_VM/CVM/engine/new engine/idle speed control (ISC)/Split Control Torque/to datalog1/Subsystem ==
  In1 : Inport
  Enable : EnablePort
  To Workspace : ToWorkspace  VariableName=datalog__engine__ISC_torque_Nm  SampleTime=-1
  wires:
  In1/1 -> To Workspace/1

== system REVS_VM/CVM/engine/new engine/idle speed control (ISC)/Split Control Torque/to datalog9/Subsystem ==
  In1 : Inport
  Enable : EnablePort
  To Workspace : ToWorkspace  VariableName=datalog__engine__ISC_est_slow_torque_Nm  SampleTime=-1
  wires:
  In1/1 -> To Workspace/1

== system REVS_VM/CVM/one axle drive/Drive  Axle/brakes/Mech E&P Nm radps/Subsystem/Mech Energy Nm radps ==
  trq_Nm : Inport
  spd_radps : Inport  Port=2
  Gain : Gain  Gain=-1
  Integrator : Integrator  ZeroCross=off
  Integrator1 : Integrator  ZeroCross=off
  Integrator2 : Integrator  ZeroCross=off
  Mux : Mux  Inputs=2
  Neg : Fcn  Expr=u(1)*(u(1) <= 0)
  Pos : Fcn  Expr=u(1)*(u(1) >= 0)
  calc_Power_kW : Fcn  Expr=u(1)*u(2)/1000
  "total_kJ " : Outport
  "pos_kJ " : Outport  Port=2
  neg_kJ : Outport  Port=3
  pwr_kW : Outport  Port=4
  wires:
  calc_Power_kW/1 -> Pos/1, Neg/1, pwr_kW/1, Integrator/1
  Gain/1 -> neg_kJ/1
  Integrator1/1 -> "pos_kJ "/1
  Integrator2/1 -> Gain/1
  Neg/1 -> Integrator2/1
  Pos/1 -> Integrator1/1
  spd_radps/1 -> Mux/2
  trq_Nm/1 -> Mux/1
  Mux/1 -> calc_Power_kW/1
  Integrator/1 -> "total_kJ "/1

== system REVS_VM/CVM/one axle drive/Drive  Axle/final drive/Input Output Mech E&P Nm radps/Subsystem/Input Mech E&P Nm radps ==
  " trq_Nm" : Inport
  spd_radps : Inport  Port=2
  iner_kgm2 : Inport  Port=3
  Compare To Constant : simulink/Logic and Bit Operations/Compare To Constant  relop=>=  const=1  OutDataTypeStr=boolean
  Constant : Constant  Value=VerboseSignal
  Subsystem : Subsystem
  pos_kJ : Outport
  neg_kJ : Outport  Port=2
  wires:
  " trq_Nm"/1 -> Subsystem/1(" trq_Nm")
  spd_radps/1 -> Subsystem/2(spd_radps)
  iner_kgm2/1 -> Subsystem/3(iner_kgm2)
  Compare To Constant/1 -> Subsystem/Enable
  Subsystem/1(pos_kJ) -> pos_kJ/1
  Subsystem/2(neg_kJ) -> neg_kJ/1
  Constant/1 -> Compare To Constant/1

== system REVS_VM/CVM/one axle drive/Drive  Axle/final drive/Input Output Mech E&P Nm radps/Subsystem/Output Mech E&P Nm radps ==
  " trq_Nm" : Inport
  spd_radps : Inport  Port=2
  iner_kgm2 : Inport  Port=3
  Compare To Constant : simulink/Logic and Bit Operations/Compare To Constant  relop=>=  const=1  OutDataTypeStr=boolean
  Constant : Constant  Value=VerboseSignal
  Subsystem : Subsystem
  pos_kJ : Outport
  neg_kJ : Outport  Port=2
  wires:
  " trq_Nm"/1 -> Subsystem/1(" trq_Nm")
  spd_radps/1 -> Subsystem/2(spd_radps)
  iner_kgm2/1 -> Subsystem/3(iner_kgm2)
  Compare To Constant/1 -> Subsystem/Enable
  Subsystem/1(pos_kJ) -> pos_kJ/1
  Subsystem/2(neg_kJ) -> neg_kJ/1
  Constant/1 -> Compare To Constant/1

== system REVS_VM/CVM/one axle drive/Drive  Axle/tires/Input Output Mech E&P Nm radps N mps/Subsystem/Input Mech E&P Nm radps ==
  " trq_Nm" : Inport
  spd_radps : Inport  Port=2
  iner_kgm2 : Inport  Port=3
  Compare To Constant : simulink/Logic and Bit Operations/Compare To Constant  relop=>=  const=1  OutDataTypeStr=boolean
  Constant : Constant  Value=VerboseSignal
  Subsystem : Subsystem
  pos_kJ : Outport
  neg_kJ : Outport  Port=2
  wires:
  Constant/1 -> Compare To Constant/1
  Subsystem/2(neg_kJ) -> neg_kJ/1
  Subsystem/1(pos_kJ) -> pos_kJ/1
  Compare To Constant/1 -> Subsystem/Enable
  iner_kgm2/1 -> Subsystem/3(iner_kgm2)
  spd_radps/1 -> Subsystem/2(spd_radps)
  " trq_Nm"/1 -> Subsystem/1(" trq_Nm")

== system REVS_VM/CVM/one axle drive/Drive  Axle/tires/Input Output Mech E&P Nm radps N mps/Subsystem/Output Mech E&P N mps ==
  force_N : Inport
  spd_mps : Inport  Port=2
  mass_kg : Inport  Port=3
  Compare To Constant : simulink/Logic and Bit Operations/Compare To Constant  relop=>=  const=1  OutDataTypeStr=boolean
  Constant : Constant  Value=VerboseSignal
  Subsystem : Subsystem
  pos_kJ : Outport
  neg_kJ : Outport  Port=2
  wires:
  Subsystem/2(neg_kJ) -> neg_kJ/1
  Subsystem/1(pos_kJ) -> pos_kJ/1
  force_N/1 -> Subsystem/1(force_N)
  spd_mps/1 -> Subsystem/2(spd_mps)
  mass_kg/1 -> Subsystem/3(mass_kg)
  Compare To Constant/1 -> Subsystem/Enable
  Constant/1 -> Compare To Constant/1

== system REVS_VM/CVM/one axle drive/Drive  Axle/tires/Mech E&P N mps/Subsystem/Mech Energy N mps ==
  force_N : Inport
  spd_mps : Inport  Port=2
  Gain : Gain  Gain=-1
  Integrator : Integrator  ZeroCross=off
  Integrator1 : Integrator  ZeroCross=off
  Integrator2 : Integrator  ZeroCross=off
  Mux : Mux  Inputs=2
  Neg : Fcn  Expr=u(1)*(u(1) <= 0)
  Pos : Fcn  Expr=u(1)*(u(1) >= 0)
  calc_Power_kW : Fcn  Expr=u(1)*u(2)/1000
  "total_kJ " : Outport
  "pos_kJ " : Outport  Port=2
  neg_kJ : Outport  Port=3
  pwr_kW : Outport  Port=4
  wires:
  calc_Power_kW/1 -> Pos/1, Neg/1, pwr_kW/1, Integrator/1
  Gain/1 -> neg_kJ/1
  Integrator1/1 -> "pos_kJ "/1
  Integrator2/1 -> Gain/1
  Neg/1 -> Integrator2/1
  Pos/1 -> Integrator1/1
  Integrator/1 -> "total_kJ "/1
  Mux/1 -> calc_Power_kW/1
  force_N/1 -> Mux/1
  spd_mps/1 -> Mux/2

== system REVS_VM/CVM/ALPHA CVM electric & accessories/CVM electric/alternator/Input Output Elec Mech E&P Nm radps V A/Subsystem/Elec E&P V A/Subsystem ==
  volts_V : Inport
  curr_A : Inport  Port=2
  Enable : EnablePort  ZeroCross=off
  Elec Energy V A : Subsystem  TreatAsAtomicUnit=on
  amps_to_workspace : ToWorkspace  VariableName=audit__elec__alternator__input_Amps  SampleTime=-1
  energy_to_workspace : ToWorkspace  VariableName=audit__elec__alternator__input_kJ  SampleTime=-1
  neg_energy_to_workspace : ToWorkspace  VariableName=audit__elec__alternator__input_neg_kJ  SampleTime=-1
  pos_energy_to_workspace : ToWorkspace  VariableName=audit__elec__alternator__input_pos_kJ  SampleTime=-1
  power_to_workspace : ToWorkspace  VariableName=audit__elec__alternator__input_kW  SampleTime=-1
  volts_to_workspace : ToWorkspace  VariableName=audit__elec__alternator__input_Volts  SampleTime=-1
  pos_kJ : Outport  InitialOutput=0
  neg_kJ : Outport  Port=2  InitialOutput=0
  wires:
  Elec Energy V A/3(neg_kJ) -> neg_kJ/1, neg_energy_to_workspace/1
  Elec Energy V A/4(pwr_kW) -> power_to_workspace/1
  Elec Energy V A/2("pos_kJ ") -> pos_kJ/1, pos_energy_to_workspace/1
  Elec Energy V A/1("total_kJ ") -> energy_to_workspace/1
  volts_V/1 -> volts_to_workspace/1, Elec Energy V A/1(volts_V)
  curr_A/1 -> amps_to_workspace/1, Elec Energy V A/2(curr_A)

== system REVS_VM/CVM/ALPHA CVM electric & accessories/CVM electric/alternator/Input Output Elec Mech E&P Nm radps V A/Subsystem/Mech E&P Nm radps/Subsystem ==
  " trq_Nm" : Inport
  spd_radps : Inport  Port=2
  iner_kgm2 : Inport  Port=3
  Enable : EnablePort  ZeroCross=off
  KE_to_workspace : ToWorkspace  VariableName=audit__mech__alternator__output_KE_kJ  SampleTime=-1
  Mech Energy Nm radps : Subsystem  TreatAsAtomicUnit=on
  Mult : Product  Inputs=**
  Square : Math  Operator=square
  energy_to_workspace : ToWorkspace  VariableName=audit__mech__alternator__output_kJ  SampleTime=-1
  inertia_to_workspace : ToWorkspace  VariableName=audit__mech__alternator__output_kgm2  SampleTime=-1
  neg_energy_to_workspace : ToWorkspace  VariableName=audit__mech__alternator__output_neg_kJ  SampleTime=-1
  one half : Gain  Gain=0.5/1000
  pos_energy_to_workspace : ToWorkspace  VariableName=audit__mech__alternator__output_pos_kJ  SampleTime=-1
  power_to_workspace : ToWorkspace  VariableName=audit__mech__alternator__output_kW  SampleTime=-1
  speed_to_workspace : ToWorkspace  VariableName=audit__mech__alternator__output_radps  SampleTime=-1
  torque_to_workspace : ToWorkspace  VariableName=audit__mech__alternator__output_Nm  SampleTime=-1
  pos_kJ : Outport  InitialOutput=0
  neg_kJ : Outport  Port=2  InitialOutput=0
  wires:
  Mult/1 -> one half/1
  Square/1 -> Mult/1
  one half/1 -> KE_to_workspace/1
  Mech Energy Nm radps/4(pwr_kW) -> power_to_workspace/1
  Mech Energy Nm radps/1("total_kJ ") -> energy_to_workspace/1
  iner_kgm2/1 -> inertia_to_workspace/1, Mult/2
  spd_radps/1 -> Mech Energy Nm radps/2(spd_radps), speed_to_workspace/1, Square/1
  " trq_Nm"/1 -> Mech Energy Nm radps/1(trq_Nm), torque_to_workspace/1
  Mech Energy Nm radps/2("pos_kJ ") -> pos_kJ/1, pos_energy_to_workspace/1
  Mech Energy Nm radps/3(neg_kJ) -> neg_energy_to_workspace/1, neg_kJ/1

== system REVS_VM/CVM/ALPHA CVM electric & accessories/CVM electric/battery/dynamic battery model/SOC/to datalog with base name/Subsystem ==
  Var : Inport
  Enable : EnablePort
  To Workspace : ToWorkspace  VariableName=datalog__battery__SoC_norm  SampleTime=-1
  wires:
  Var/1 -> To Workspace/1

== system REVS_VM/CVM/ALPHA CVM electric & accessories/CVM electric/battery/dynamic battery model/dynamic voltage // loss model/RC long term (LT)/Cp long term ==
  bus_in : Inport
  Bus Selector : BusSelector  OutputSignals=pack_curr_A
  Cp_LT charge : Subsystem
  Cp_LT discharge : Subsystem
  Switch : Switch
  Cp_LT_Farad : Outport
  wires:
  Switch/1 -> Cp_LT_Farad/1
  bus_in/1 -> Cp_LT charge/1(bus), Cp_LT discharge/1(bus), Bus Selector/1
  Bus Selector/1 -> Switch/2  "<pack_curr_A>"
  Cp_LT discharge/1(out) -> Switch/1
  Cp_LT charge/1(out) -> Switch/3

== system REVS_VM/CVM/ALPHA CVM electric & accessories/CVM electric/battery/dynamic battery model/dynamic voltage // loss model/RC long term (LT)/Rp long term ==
  bus_in : Inport
  Bus Selector : BusSelector  OutputSignals=pack_curr_A
  Rp_LT charge : Subsystem
  Rp_LT discharge : Subsystem
  Switch : Switch
  Rp_LT_Ohm : Outport
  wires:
  Switch/1 -> Rp_LT_Ohm/1
  Bus Selector/1 -> Switch/2  "<pack_curr_A>"
  bus_in/1 -> Rp_LT discharge/1(bus), Rp_LT charge/1(bus), Bus Selector/1
  Rp_LT discharge/1(out) -> Switch/1
  Rp_LT charge/1(out) -> Switch/3

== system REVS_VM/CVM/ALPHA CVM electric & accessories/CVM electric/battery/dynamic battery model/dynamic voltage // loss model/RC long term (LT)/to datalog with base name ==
  Var : Inport
  Constant : Constant  Value=VerboseSignal
  Constant1 : Constant  Value=VerboseLevel
  Relational Operator : RelationalOperator  OutDataTypeStr=boolean  ZeroCross=off
  Subsystem : Subsystem
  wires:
  Constant1/1 -> Relational Operator/2
  Relational Operator/1 -> Subsystem/Enable
  Constant/1 -> Relational Operator/1
  Var/1 -> Subsystem/1(Var)

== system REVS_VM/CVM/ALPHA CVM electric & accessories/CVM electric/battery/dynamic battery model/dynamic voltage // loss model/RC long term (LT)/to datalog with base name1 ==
  Var : Inport
  Constant : Constant  Value=VerboseSignal
  Constant1 : Constant  Value=VerboseLevel
  Relational Operator : RelationalOperator  OutDataTypeStr=boolean  ZeroCross=off
  Subsystem : Subsystem
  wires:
  Constant1/1 -> Relational Operator/2
  Relational Operator/1 -> Subsystem/Enable
  Constant/1 -> Relational Operator/1
  Var/1 -> Subsystem/1(Var)

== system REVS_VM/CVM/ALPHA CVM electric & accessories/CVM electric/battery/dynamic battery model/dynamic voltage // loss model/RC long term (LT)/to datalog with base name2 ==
  Var : Inport
  Constant : Constant  Value=VerboseSignal
  Constant1 : Constant  Value=VerboseLevel
  Relational Operator : RelationalOperator  OutDataTypeStr=boolean  ZeroCross=off
  Subsystem : Subsystem
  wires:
  Constant1/1 -> Relational Operator/2
  Relational Operator/1 -> Subsystem/Enable
  Constant/1 -> Relational Operator/1
  Var/1 -> Subsystem/1(Var)

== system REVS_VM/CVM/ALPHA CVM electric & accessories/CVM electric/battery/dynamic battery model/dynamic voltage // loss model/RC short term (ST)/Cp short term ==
  bus_in : Inport
  Bus Selector : BusSelector  OutputSignals=pack_curr_A
  Cp_ST charge : Subsystem
  Cp_ST discharge : Subsystem
  Switch : Switch
  Cp_ST_Farad : Outport
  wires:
  Switch/1 -> Cp_ST_Farad/1
  bus_in/1 -> Cp_ST charge/1(bus), Cp_ST discharge/1(bus), Bus Selector/1
  Bus Selector/1 -> Switch/2  "<pack_curr_A>"
  Cp_ST discharge/1(out) -> Switch/1
  Cp_ST charge/1(out) -> Switch/3

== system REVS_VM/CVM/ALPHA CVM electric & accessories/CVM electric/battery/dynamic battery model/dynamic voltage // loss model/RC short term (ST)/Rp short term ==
  bus_in : Inport
  Bus Selector : BusSelector  OutputSignals=pack_curr_A
  Rp_ST charge : Subsystem
  Rp_ST discharge : Subsystem
  Switch : Switch
  Rp_ST_Ohm : Outport
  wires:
  Switch/1 -> Rp_ST_Ohm/1
  Rp_ST discharge/1(out) -> Switch/1
  Rp_ST charge/1(out) -> Switch/3
  bus_in/1 -> Rp_ST charge/1(bus), Rp_ST discharge/1(bus), Bus Selector/1
  Bus Selector/1 -> Switch/2  "<pack_curr_A>"

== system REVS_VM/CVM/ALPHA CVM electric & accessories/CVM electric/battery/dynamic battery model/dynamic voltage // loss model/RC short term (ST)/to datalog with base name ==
  Var : Inport
  Constant : Constant  Value=VerboseSignal
  Constant1 : Constant  Value=VerboseLevel
  Relational Operator : RelationalOperator  OutDataTypeStr=boolean  ZeroCross=off
  Subsystem : Subsystem
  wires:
  Constant1/1 -> Relational Operator/2
  Relational Operator/1 -> Subsystem/Enable
  Constant/1 -> Relational Operator/1
  Var/1 -> Subsystem/1(Var)

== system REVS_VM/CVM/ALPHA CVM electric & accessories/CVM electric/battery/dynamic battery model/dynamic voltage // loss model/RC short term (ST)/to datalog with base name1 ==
  Var : Inport
  Constant : Constant  Value=VerboseSignal
  Constant1 : Constant  Value=VerboseLevel
  Relational Operator : RelationalOperator  OutDataTypeStr=boolean  ZeroCross=off
  Subsystem : Subsystem
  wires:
  Constant1/1 -> Relational Operator/2
  Relational Operator/1 -> Subsystem/Enable
  Constant/1 -> Relational Operator/1
  Var/1 -> Subsystem/1(Var)
